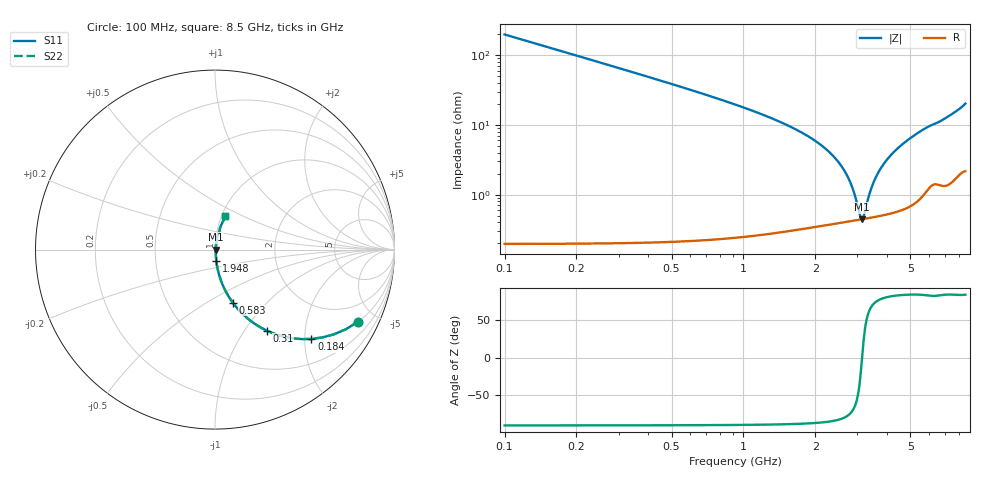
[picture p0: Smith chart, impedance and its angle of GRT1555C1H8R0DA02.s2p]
!Murata Part Number: GRT1555C1H8R0DA02
!These Parameters are Measured in Series Mode Connection
!Data Generated on Jun 19, 2026
!  o--ll--o
!Port1  Port2
!  o------o
!Operation Temp=25[degC], DC Bias Voltage=0[V]
!Freq. Start=100[MHz] Stop=9[GHz] 401[Steps]
# Hz S RI R 50
!Freq.(Hz) S11(Real) S11(Imag) S21(Real) S21(Imag) S12(Real) S12(Imag) S22(Real) S22(Imag)
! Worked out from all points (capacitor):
!   401 points, 100 MHz to 8.5 GHz, reference 50 ohm
!   read as one part in series: C = 8 pF near 142 MHz
!   lowest |Z| = 445 mohm at 3.145 GHz (marker M1)
!   series resonance near 3.139 GHz, so ESL is about 320 pH
!   S11 on the Smith chart (normalised r, x): 100 MHz: 1.00, -3.97; 184 MHz: 1.00, -2.15; 310 MHz: 1.00, -1.27; 583 MHz: 1.00, -0.66; 1.948 GHz: 1.01, -0.13; 8.5 GHz: 1.04, +0.40
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1e8  0.7977 -0.4012  0.2023 0.4012  0.2023 0.4012  0.7977 -0.4012
1.84e8  0.5371 -0.4977  0.4629 0.4977  0.4629 0.4977  0.5371 -0.4977
3.1e8  0.2882 -0.4513  0.7118 0.4513  0.7118 0.4513  0.2882 -0.4513
4.36e8  0.1679 -0.3714  0.8321 0.3714  0.8321 0.3714  0.1679 -0.3714
5.83e8  0.0994 -0.2959  0.9006 0.2959  0.9006 0.2959  0.0994 -0.2959
9.61e8  0.0361 -0.1801  0.9639 0.1801  0.9639 0.1801  0.0361 -0.1801
1.507e9  0.013 -0.0997  0.987 0.0997  0.987 0.0997  0.013 -0.0997
1.948e9  0.00725 -0.062  0.9928 0.062  0.9928 0.062  0.00725 -0.062
2.557e9  0.00461 -0.026  0.9954 0.026  0.9954 0.026  0.00461 -0.026
2.746e9  0.00438 -0.0169  0.9956 0.0169  0.9956 0.0169  0.00438 -0.0169
2.914e9  0.00432 -0.00937  0.9957 0.00937  0.9957 0.00937  0.00432 -0.00937
3.082e9  0.00438 -0.0023  0.9956 0.0023  0.9956 0.0023  0.00438 -0.0023
3.145e9  0.00443 0.000262  0.9956 -0.000262  0.9956 -0.000262  0.00443 0.000262
3.208e9  0.00449 0.00277  0.9955 -0.00277  0.9955 -0.00277  0.00449 0.00277
3.418e9  0.00477 0.0108  0.9952 -0.0108  0.9952 -0.0108  0.00477 0.0108
3.607e9  0.00514 0.0178  0.9949 -0.0178  0.9949 -0.0178  0.00514 0.0178
3.901e9  0.00588 0.028  0.9941 -0.028  0.9941 -0.028  0.00588 0.028
4.3e9  0.00724 0.0412  0.9928 -0.0412  0.9928 -0.0412  0.00724 0.0412
4.909e9  0.0102 0.0605  0.9898 -0.0605  0.9898 -0.0605  0.0102 0.0605
5.707e9  0.0172 0.0846  0.9828 -0.0846  0.9828 -0.0846  0.0172 0.0846
7.114e9  0.0289 0.1229  0.9711 -0.1229  0.9711 -0.1229  0.0289 0.1229
8.5e9  0.058 0.1859  0.942 -0.1859  0.942 -0.1859  0.058 0.1859
